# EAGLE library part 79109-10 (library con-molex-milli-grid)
RECEPTACAL
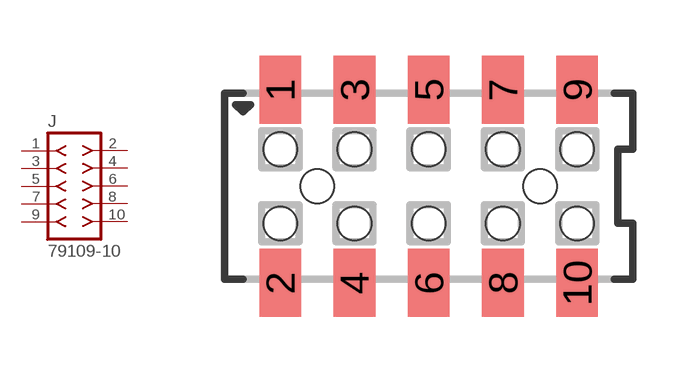
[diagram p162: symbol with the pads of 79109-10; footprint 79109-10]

Designator prefix J

## 79109-10  [79109-10]
1  1  pas
2  2  pas
3  3  pas
4  4  pas
5  5  pas
6  6  pas
7  7  pas
8  8  pas
9  9  pas
10  10  pas

## Footprint 79109-10 (pad centres in mm)
RECEPTACAL SMD Dual Row, Vertical, Pass-Thru
smd 1.12 x 1.83: 1 -4,2.6; 2 -4,-2.6; 3 -2,2.6; 4 -2,-2.6; 5 0,2.6; 6 0,-2.6; 7 2,2.6; 8 2,-2.6; 9 4,2.6; 10 4,-2.6
hole 0.914 at -3,0
hole 0.914 at -4,1
hole 0.914 at -4,-1
hole 0.914 at -2,-1
hole 0.914 at -2,1
hole 0.914 at 0,-1
hole 0.914 at 0,1
hole 0.914 at 3,0
hole 0.914 at 2,1
hole 0.914 at 2,-1
hole 0.914 at 4,1
hole 0.914 at 4,-1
